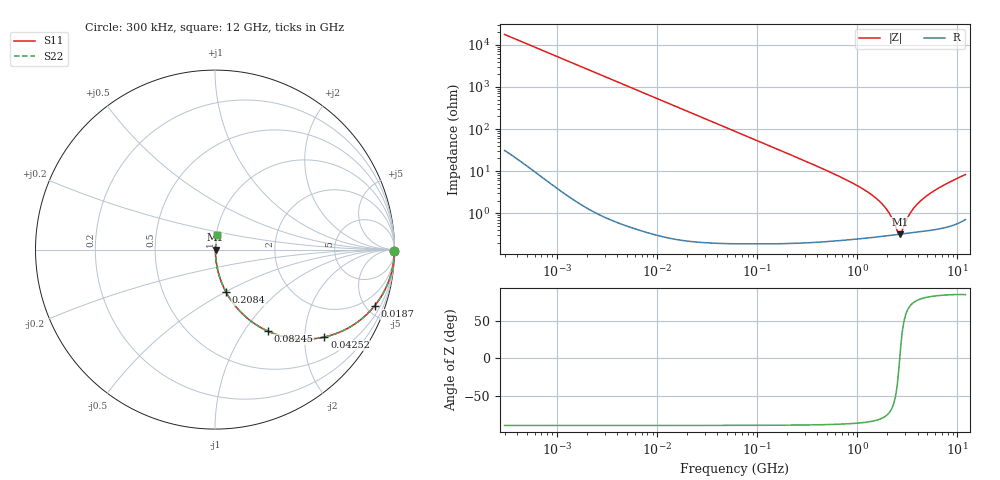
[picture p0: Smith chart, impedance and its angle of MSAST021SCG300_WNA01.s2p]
! MSAST021SCG300_WNA01  S-PARAMETER MODEL  ( Standard Model )
! Model Generated by TAIYO YUDEN Corporation (http://www.ty-top.com)
! Version 2.0
! TAIYO YUDEN Control No. 231201
! Copyright(c) 2023 TAIYO YUDEN CO.,LTD. All Rights Reserved.
! Product Description (link to TY-COMPAS)
! https://ds.yuden.co.jp/TYCOMPAS/or/detail?pn=MSAST021SCG300JWNA01&u=M
! Products Name : Multilayer Ceramic Capacitors
! Characteristics :
!  Capacitance : 30 [pF] , Rated Voltage : 25 [V] , TCC : CG / C0G
!  Case Size : 0.25 x 0.125 / 0.0098 x 0.0049 [mm/inch] , Thickness : 0.125 / 0.0049 [mm/inch]
!  (Conditions: Temperature = 25 [degC] , DC Bias Voltage = 0 [V])
! External Node Assignments :
!  1  o---| |---o  2
! GND o---------o GND
! Frequency Range : 0.3MHz  -  12000MHz  [ 401 STEP ]
# MHZ S RI R 50
! Freq[MHz].  S11 Real  S11 Imag  S21 Real  S21 Imag  S12 Real  S12 Imag  S22 Real  S22 Imag
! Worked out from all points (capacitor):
!   401 points, 300 kHz to 12 GHz, reference 50 ohm
!   read as one part in series: C = 30 pF near 316.3 kHz
!   lowest |Z| = 317 mohm at 2.651 GHz (marker M1)
!   series resonance near 2.651 GHz, so ESL is about 120 pH
!   S11 on the Smith chart (normalised r, x): 300 kHz: open; 18.7 MHz: 1.00, -5.68; 42.52 MHz: 1.00, -2.50; 82.45 MHz: 1.00, -1.29; 208.4 MHz: 1.00, -0.51; 12 GHz: 1.01, +0.17
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0.3  1 -0.00566  4.19e-05 0.00566  4.19e-05 0.00566  1 -0.00566
1.769972  0.9989 -0.0333  0.00113 0.0333  0.00113 0.0333  0.9989 -0.0333
4.84353  0.9917 -0.0905  0.00829 0.0905  0.00829 0.0905  0.9917 -0.0905
10.44266  0.9627 -0.1893  0.0373 0.1893  0.0373 0.1893  0.9627 -0.1893
18.70358  0.8895 -0.3132  0.1105 0.3132  0.1105 0.3132  0.8895 -0.3132
27.82928  0.7843 -0.4108  0.2157 0.4108  0.2157 0.4108  0.7843 -0.4108
42.51912  0.6091 -0.4872  0.3909 0.4872  0.3909 0.4872  0.6091 -0.4872
60  0.4392 -0.4952  0.5608 0.4952  0.5608 0.4952  0.4392 -0.4952
82.45425  0.2933 -0.4538  0.7067 0.4538  0.7067 0.4538  0.2933 -0.4538
129.3602  0.1447 -0.3495  0.8553 0.3495  0.8553 0.3495  0.1447 -0.3495
208.3979  0.0618 -0.237  0.9382 0.237  0.9382 0.237  0.0618 -0.237
353.9943  0.023 -0.1434  0.977 0.1434  0.977 0.1434  0.023 -0.1434
1197.383  0.00375 -0.0347  0.9963 0.0347  0.9963 0.0347  0.00375 -0.0347
1645.489  0.00314 -0.0194  0.9969 0.0194  0.9969 0.0194  0.00314 -0.0194
2088.533  0.00304 -0.0094  0.997 0.0094  0.997 0.0094  0.00304 -0.0094
2514.07  0.00312 -0.00206  0.9969 0.00206  0.9969 0.00206  0.00312 -0.00206
2650.866  0.00316 1.13e-06  0.9968 -1.13e-06  0.9968 -1.13e-06  0.00316 1.13e-06
2795.104  0.00322 0.00206  0.9968 -0.00206  0.9968 -0.00206  0.00322 0.00206
3454.93  0.00352 0.0104  0.9965 -0.0104  0.9965 -0.0104  0.00352 0.0104
4385.161  0.00407 0.0202  0.9959 -0.0202  0.9959 -0.0202  0.00407 0.0202
6699.894  0.00594 0.0408  0.9941 -0.0408  0.9941 -0.0408  0.00594 0.0408
12000  0.0137 0.081  0.9863 -0.081  0.9863 -0.081  0.0137 0.081
